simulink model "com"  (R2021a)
settings: Solver=FixedStepDiscrete  StartTime=0.0  StopTime=Inf  RelTol=1e-3  EnableMultiTasking=on
undefined symbols (not defined in the file): A, ADCIN0, ADCIN1, ADCINA0, ADCINB0, bit, Compare, conversion, DCAEVT1, DCAEVT1FILT, Digital, Down, ended, Event, Filtered, GPTRIP1SEL, GPTRIP2SEL, input, Module, of, Single, start, Trip, TZ1, TZ2, Up, version, Zone
libraries: c2802xlib x3, c280xlib x2

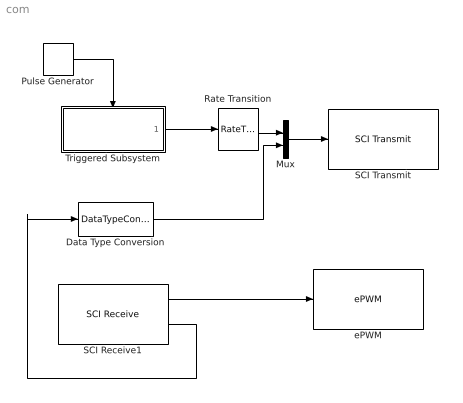
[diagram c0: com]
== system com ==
  Data Type Conversion : DataTypeConversion  OutDataTypeStr=single
  Mux : Mux  Inputs=2
  Pulse Generator : DiscretePulseGenerator  SampleTime=1e-4
  Rate Transition : RateTransition  OutPortSampleTime=0.1
  SCI Receive1 : c280xlib/SCI Receive  sciModule=A  dataHead='S'  dataTail='E'  dataType=single  dataDim=1  initValue=0  errOption=Output the last received value  errValue=0  sampleTime=0.1  outputStatus=on  postInterrupt=off  numFifo=1
  SCI Transmit : c280xlib/SCI Transmit  sciModule=A  dataHead='S'  dataTail='E'  postInterrupt=off  numFifo=1
  Triggered Subsystem : Subsystem  TreatAsAtomicUnit=on
  ePWM : c2802xlib/ePWM  PwmType=C2000  useModule=ePWM5  ePWMxLINKTBPRD=Not Linked  periodUnits=Clock cycles  timerSource=Specify via dialog  timerPeriod_clk=64000  timerPeriod_sec=0.0001  tbshadow=Counter equals to zero  countingMode=Up-Down  phaseActiveEnable=Disable  phaseDirection=Count down after sync  phaseActive=0  synchronizationEnable=off  dcaevt1Sync=off  dcbevt1Sync=off  synchronizationOption=Disable  perSynchronizationOption=Counter equals to period (CTR=PRD)  clockPrescale=1  HSclockPrescale=1  enswap=off  ePWMxAStatus=on  ePWMxAactionLogic1=Do nothing  ePWMxAactionLogic2=Do nothing  ePWMxAactionLogic3=Clear  ePWMxAactionLogic4=Set  ePWMxAactionLogic5=Do nothing  ePWMxAactionLogic6=Do nothing  ePWMxACSFenable=off  ePWMxACSFvalue=Forcing disable  ePWMxASFreload=Zero  ePWMxBStatus=off  ePWMxBactionLogic1=Set  ePWMxBactionLogic2=Clear  ePWMxBactionLogic3=Do nothing  ePWMxBactionLogic4=Do nothing  ePWMxBactionLogic5=Clear  ePWMxBactionLogic6=Set  ePWMxBCSFenable=off  ePWMxBCSFvalue=Forcing disable  ePWMxBSFreload=Zero  ePWNxBOutWay=off  ePWMxLINKCMPA=Not Linked  CMPAUnits=Percentages  CMPASource=Input port  CMPAValue_per=0  CMPAValue_clk=32000  enCMPAshadow=Counter equals to zero (CTR=Zero)  ePWMxLINKCMPB=Not Linked  CMPBUnits=Clock cycles  CMPBSource=Specify via dialog  CMPBValue_per=50  CMPBValue_clk=32000  enCMPBshadow=Counter equals to zero (CTR=Zero)  ePWMxLINKCMPC=Not Linked  CMPCUnits=Clock cycles  CMPCSource=Specify via dialog  CMPCValue_per=50  CMPCValue_clk=32000  enCMPCshadow=Counter equals to zero (CTR=Zero)  ePWMxLINKCMPD=Not Linked  CMPDUnits=Clock cycles  CMPDSource=Specify via dialog  CMPDValue_per=50  CMPDValue_clk=32000  enCMPDshadow=Counter equals to zero (CTR=Zero)  enableDBePWMxA=off  enableDBePWMxB=off  enhalfcycle=off  DBpolarity=Active high (AH)  DBedgeDelay=Positive  DBSource_ePWMxA=ePWMxA  DBSource_ePWMxB=ePWMxA  DBPeriodUnits=Clock cycles  DBperiodSource=Specify via dialog  REDperiod=0  FEDperiod=0  REDperiod_sec=0  FEDperiod_sec=0  LoadModeDBRED=Immediate without using shadow  LoadModeDBFED=Immediate without using shadow  adcstartModuleA=off  adcrequestEventA=First event  adcstartEventA=Counter equals to zero (CTR=Zero)  adcstartEventA_type2=Digital Compare Module A Event 1 start of conversion (DCAEVT1.soc)  adcstartModuleB=off  adcrequestEventB=First event  adcstartEventB=Counter equals to zero (CTR=Zero)  adcstartEventB_type2=Counter equals to zero (CTR=Zero)  intEn=off  intPrd=First event  intSel=Counter equals to zero (CTR=Zero)  intSel_type2=Counter equals to zero (CTR=Zero)  hrpe=off  enHRPWM=off  HRPWM_LoadMode=Counter equals to period (CTR=PRD)  HRPWM_CTLMode=Duty or Period control mode  HRPWM_EDGMode=Both edge  hrpeb=off  enHRPWMB=off  HRPWM_LoadModeB=Counter equals to zero (CTR=ZERO)  HRPWM_CTLModeB=Duty or Period control mode  HRPWM_EDGModeB=Both edge  enHRDBRED=off  enHRDBFED=off  enSFO=on  enautoconv=on  chopperEnable=off  chopperFrequency=1  chopperFirstwidth=1  chopperDuty=12.5%  tripZonesource=Specify via dialog  tzselOSHT1=off  tzselOSHT2=off  tzselOSHT3=off  tzselOSHDCAEV1=off  tzselOSHDCBEV1=off  tzselCBC1=off  tzselCBC2=off  tzselCBC3=off  tzselCBCDCAEV2=off  tzselCBCDCBEV2=off  tzselOSHT4=off  tzselOSHT5=off  tzselOSHT6=off  tzselCBC4=off  tzselCBC5=off  tzselCBC6=off  enTzOstIntr=off  enTzCbcIntr=off  enTzDCAEVT1Intr=off  enTzDCAEVT2Intr=off  enTzDCBEVT1Intr=off  enTzDCBEVT2Intr=off  ePWMxAforced=No action  ePWMxBforced=No action  DCAEVT1forced=No action  DCBEVT1forced=No action  DCAEVT2forced=No action  DCBEVT2forced=No action  dcah=Trip Zone 1 input (TZ1)  dcal=Trip Zone 1 input (TZ1)  dcbh=Trip Zone 1 input (TZ1)  dcbl=Trip Zone 1 input (TZ1)  dcah_type2=GPTRIP1SEL/(TZ1)  dcal_type2=GPTRIP2SEL/(TZ2)  dcbh_type2=GPTRIP1SEL/(TZ1)  dcbl_type2=GPTRIP2SEL/(TZ2)  gendcaevt1=Event disabled  gendcaevt2=Event disabled  gendcbevt1=Event disabled  gendcbevt2=Event disabled  dcaevt1src=DCAEVT1 with sync  dcaevt2src=DCAEVT2 with sync  dcbevt1src=DCBEVT1 with sync  dcbevt2src=DCBEVT2 with sync  pulsesel=Counter equals to zero (CTR=Zero)  blankinv=off  blankoffset=0  blankwidth=0  evsrcsel=Filtered version of DCAEVT1 (DCAEVT1FILT)  encape=off
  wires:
  Pulse Generator/1 -> Triggered Subsystem/Trigger
  Triggered Subsystem/1(Out1) -> Rate Transition/1
  SCI Receive1/1 -> ePWM/1
  Rate Transition/1 -> Mux/1
  Mux/1 -> SCI Transmit/1
  SCI Receive1/2 -> Data Type Conversion/1
  Data Type Conversion/1 -> Mux/2

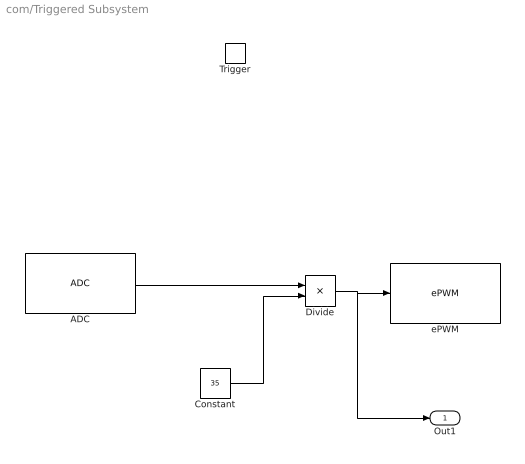
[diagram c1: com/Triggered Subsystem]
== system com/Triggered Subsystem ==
  Trigger : TriggerPort  VariantControl=(inherit)
  ADC : c2802xlib/ADC  blkParamProc=C2000  ADCModule=1  samplingMode=Single sample mode  ADCResolution=12-bit (Single-ended input)  useSOC1=SOC0  useSOC2=SOC0_SOC1  SOCAcquisitionWindow=7  SOCTriggerSource=Software  SOCInterruptTrigger=No ADCINT  Ts=-1  dType=single  postInterrupt=off  interruptSel=ADCINT1  ADCINTContinuous=off  endma=off  chdma=1  conv1=ADCINA6  conv2=ADCINA0 and ADCINB0  conv1_Type4=ADCIN0  conv2_Type4=ADCIN0 and ADCIN1
  Constant : Constant  Value=35  OutDataTypeStr=single
  Divide : Product  Inputs=*/
  ePWM : c2802xlib/ePWM  PwmType=C2000  useModule=ePWM4  ePWMxLINKTBPRD=Not Linked  periodUnits=Clock cycles  timerSource=Specify via dialog  timerPeriod_clk=64000  timerPeriod_sec=0.0001  tbshadow=Counter equals to zero  countingMode=Up-Down  phaseActiveEnable=Disable  phaseDirection=Count down after sync  phaseActive=0  synchronizationEnable=off  dcaevt1Sync=off  dcbevt1Sync=off  synchronizationOption=Disable  perSynchronizationOption=Counter equals to period (CTR=PRD)  clockPrescale=1  HSclockPrescale=1  enswap=off  ePWMxAStatus=on  ePWMxAactionLogic1=Do nothing  ePWMxAactionLogic2=Do nothing  ePWMxAactionLogic3=Clear  ePWMxAactionLogic4=Set  ePWMxAactionLogic5=Do nothing  ePWMxAactionLogic6=Do nothing  ePWMxACSFenable=off  ePWMxACSFvalue=Forcing disable  ePWMxASFreload=Zero  ePWMxBStatus=off  ePWMxBactionLogic1=Set  ePWMxBactionLogic2=Clear  ePWMxBactionLogic3=Do nothing  ePWMxBactionLogic4=Do nothing  ePWMxBactionLogic5=Clear  ePWMxBactionLogic6=Set  ePWMxBCSFenable=off  ePWMxBCSFvalue=Forcing disable  ePWMxBSFreload=Zero  ePWNxBOutWay=off  ePWMxLINKCMPA=Not Linked  CMPAUnits=Percentages  CMPASource=Input port  CMPAValue_per=0  CMPAValue_clk=32000  enCMPAshadow=Counter equals to zero (CTR=Zero)  ePWMxLINKCMPB=Not Linked  CMPBUnits=Clock cycles  CMPBSource=Specify via dialog  CMPBValue_per=50  CMPBValue_clk=32000  enCMPBshadow=Counter equals to zero (CTR=Zero)  ePWMxLINKCMPC=Not Linked  CMPCUnits=Clock cycles  CMPCSource=Specify via dialog  CMPCValue_per=50  CMPCValue_clk=32000  enCMPCshadow=Counter equals to zero (CTR=Zero)  ePWMxLINKCMPD=Not Linked  CMPDUnits=Clock cycles  CMPDSource=Specify via dialog  CMPDValue_per=50  CMPDValue_clk=32000  enCMPDshadow=Counter equals to zero (CTR=Zero)  enableDBePWMxA=off  enableDBePWMxB=off  enhalfcycle=off  DBpolarity=Active high (AH)  DBedgeDelay=Positive  DBSource_ePWMxA=ePWMxA  DBSource_ePWMxB=ePWMxA  DBPeriodUnits=Clock cycles  DBperiodSource=Specify via dialog  REDperiod=0  FEDperiod=0  REDperiod_sec=0  FEDperiod_sec=0  LoadModeDBRED=Immediate without using shadow  LoadModeDBFED=Immediate without using shadow  adcstartModuleA=off  adcrequestEventA=First event  adcstartEventA=Counter equals to zero (CTR=Zero)  adcstartEventA_type2=Digital Compare Module A Event 1 start of conversion (DCAEVT1.soc)  adcstartModuleB=off  adcrequestEventB=First event  adcstartEventB=Counter equals to zero (CTR=Zero)  adcstartEventB_type2=Counter equals to zero (CTR=Zero)  intEn=off  intPrd=First event  intSel=Counter equals to zero (CTR=Zero)  intSel_type2=Counter equals to zero (CTR=Zero)  hrpe=off  enHRPWM=off  HRPWM_LoadMode=Counter equals to period (CTR=PRD)  HRPWM_CTLMode=Duty or Period control mode  HRPWM_EDGMode=Both edge  hrpeb=off  enHRPWMB=off  HRPWM_LoadModeB=Counter equals to zero (CTR=ZERO)  HRPWM_CTLModeB=Duty or Period control mode  HRPWM_EDGModeB=Both edge  enHRDBRED=off  enHRDBFED=off  enSFO=on  enautoconv=on  chopperEnable=off  chopperFrequency=1  chopperFirstwidth=1  chopperDuty=12.5%  tripZonesource=Specify via dialog  tzselOSHT1=off  tzselOSHT2=off  tzselOSHT3=off  tzselOSHDCAEV1=off  tzselOSHDCBEV1=off  tzselCBC1=off  tzselCBC2=off  tzselCBC3=off  tzselCBCDCAEV2=off  tzselCBCDCBEV2=off  tzselOSHT4=off  tzselOSHT5=off  tzselOSHT6=off  tzselCBC4=off  tzselCBC5=off  tzselCBC6=off  enTzOstIntr=off  enTzCbcIntr=off  enTzDCAEVT1Intr=off  enTzDCAEVT2Intr=off  enTzDCBEVT1Intr=off  enTzDCBEVT2Intr=off  ePWMxAforced=No action  ePWMxBforced=No action  DCAEVT1forced=No action  DCBEVT1forced=No action  DCAEVT2forced=No action  DCBEVT2forced=No action  dcah=Trip Zone 1 input (TZ1)  dcal=Trip Zone 1 input (TZ1)  dcbh=Trip Zone 1 input (TZ1)  dcbl=Trip Zone 1 input (TZ1)  dcah_type2=GPTRIP1SEL/(TZ1)  dcal_type2=GPTRIP2SEL/(TZ2)  dcbh_type2=GPTRIP1SEL/(TZ1)  dcbl_type2=GPTRIP2SEL/(TZ2)  gendcaevt1=Event disabled  gendcaevt2=Event disabled  gendcbevt1=Event disabled  gendcbevt2=Event disabled  dcaevt1src=DCAEVT1 with sync  dcaevt2src=DCAEVT2 with sync  dcbevt1src=DCBEVT1 with sync  dcbevt2src=DCBEVT2 with sync  pulsesel=Counter equals to zero (CTR=Zero)  blankinv=off  blankoffset=0  blankwidth=0  evsrcsel=Filtered version of DCAEVT1 (DCAEVT1FILT)  encape=off
  Out1 : Outport
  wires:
  Divide/1 -> Out1/1, ePWM/1
  Constant/1 -> Divide/2
  ADC/1 -> Divide/1
